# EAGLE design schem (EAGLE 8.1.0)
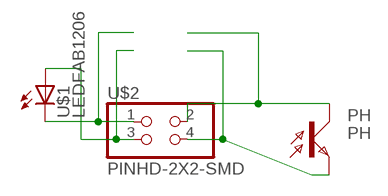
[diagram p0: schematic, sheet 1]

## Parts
PH  PH  PHOTOTRANSISTOR-NPN1206  [OP1206]
U$1  LEDFAB1206  [LED1206FAB]
U$2  PINHD-2X2-SMD  [2X02SMD]

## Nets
N$1: U$1.1(A) U$2.3
N$2: U$1.2(C) U$2.1
N$3: PH.EMITTER(E) U$2.4
N$4: PH.COLLECTOR(C) U$2.2

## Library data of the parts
PH = fab:PHOTOTRANSISTOR-NPN
U$1 = fab:LED: LED
U$2 = fab:PINHD-2X2-SMD

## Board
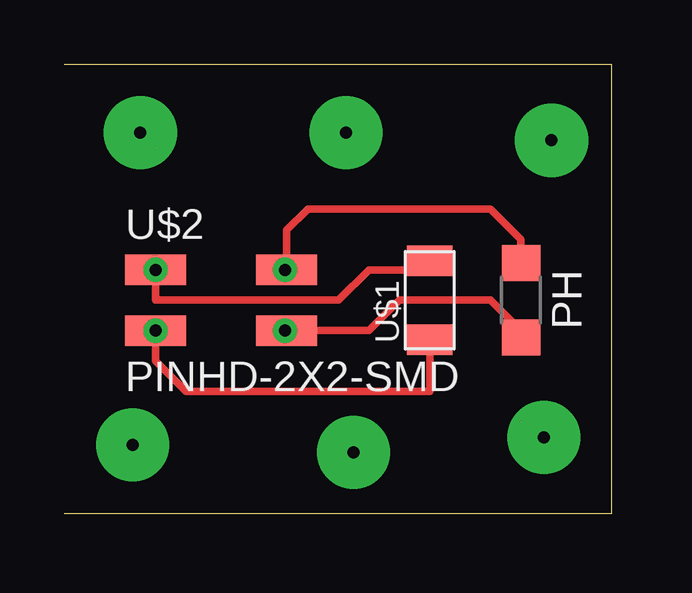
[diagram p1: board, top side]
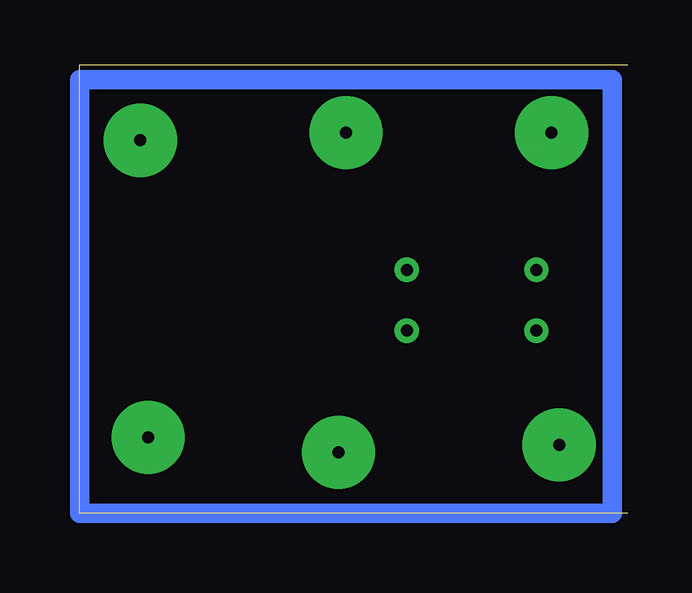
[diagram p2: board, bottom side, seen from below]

Size 22.84 x 18.72 mm. Coordinates in mm from the lower left corner, seen from the top.
Outline: 0,0 22.84,0 22.84,18.72 0,18.72
Copper layers (1*16): Top 0.035mm / dielectric 1.5mm / Bottom 0.035mm
Design rules "default": minimum track width 10mil, minimum drill 24mil, track to track 8mil, track to pad 8mil, pad to pad 8mil, via to via 8mil, smd to smd 8mil, copper to edge 40mil, drill to drill 8mil, minimum pad ring 10mil, minimum via ring 8mil, stop-mask expansion 4mil, vias tented up to drill 0mil, thermal gap 10mil

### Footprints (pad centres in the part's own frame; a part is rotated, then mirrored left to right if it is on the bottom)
OP1206 = smd 1.5 x 1.6: COLLECTOR -1.55,0; EMITTER 1.55,0
LED1206FAB = smd 1.27 x 1.905: 1 -1.651,0; 2 1.651,0
2X02SMD = smd 2.54 x 1.27: 1 -2.54,1.27; 2 2.92,1.27; 3 -2.54,-1.27; 4 2.92,-1.27

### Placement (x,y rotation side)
PH  19.05,8.89 270 top
U$1  15.24,8.89 90 top
U$2  6.35,8.89 0 top

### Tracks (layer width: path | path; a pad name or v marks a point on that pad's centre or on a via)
N$1  (via drill 0.5 pad 1.02)
  Top 0.305: U$2.3 3.81,6.35 5.08,5.08 15.24,5.08 U$1.1
  other vias: 3.81,7.62
N$2  (via drill 0.5 pad 1.02)
  Top 0.305: U$2.1 3.81,8.89 11.43,8.89 12.7,10.16 14.86,10.16 U$1.2
  other vias: 3.81,10.16
N$3
  Top 0.305: PH.EMITTER 19.05,7.62 17.78,8.89 13.97,8.89 12.7,7.62 U$2.4
N$4
  Top 0.305: U$2.2 9.27,11.81 10.16,12.7 17.78,12.7 19.05,11.43 PH.COLLECTOR
N$5  (1 unrouted)
N$6  (1 unrouted)
N$7
  Bottom 0.813: 0.64,18.1 22.86,18.1 22.86,0 0.64,0 0.64,18.1
N$8  (via drill 0.5 pad 3.05)
  other vias: 3.18,15.88
N$9  (via drill 0.5 pad 3.05)
  other vias: 20,3.17
N$10  (via drill 0.5 pad 3.05)
  other vias: 11.75,15.88
N$11  (via drill 0.5 pad 3.05)
  other vias: 12.06,2.54
N$12  (via drill 0.5 pad 3.05)
  other vias: 2.86,2.86
N$13  (via drill 0.5 pad 3.05)
  other vias: 20.32,15.56
N$14  (via drill 0.5 pad 1.02)
  other vias: 9.21,10.16
N$15  (via drill 0.5 pad 1.02)
  other vias: 9.21,7.62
